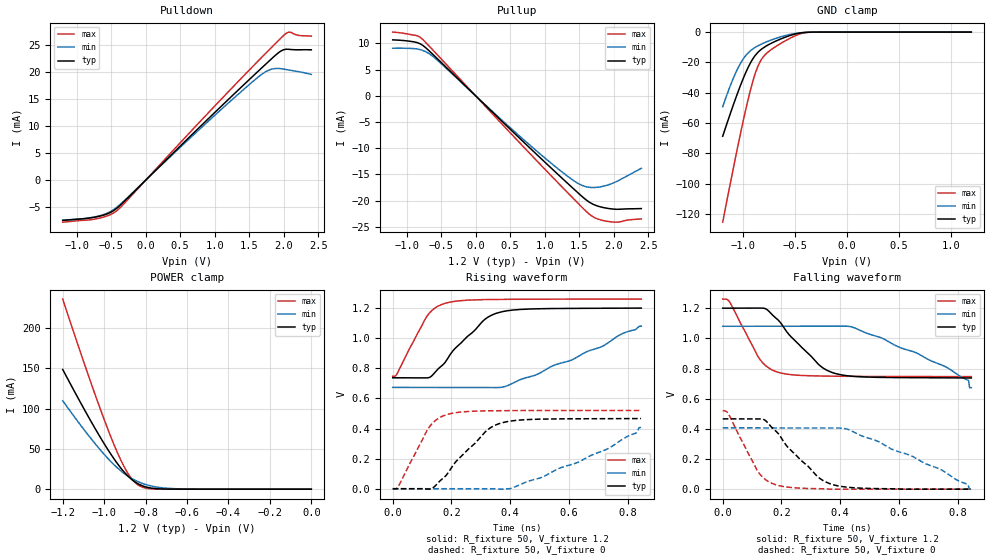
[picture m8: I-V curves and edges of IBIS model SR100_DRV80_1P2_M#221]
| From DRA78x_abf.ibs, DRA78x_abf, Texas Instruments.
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| Model based on original model for DDR_DIFFIOPB_V
|   Sub model SR100_DRV80_1P2
[model]   SR100_DRV80_1P2_M#221
|[Description]  [1.2V-I/O-X-X]
|   , ,
|[Input Load]
|[Output Drive]
|Voltage   1.2V
|Mode   I/O
Model_type   I/O
Polarity   Non-Inverting
Enable   Active-Low
Vinl =  0.47
Vinh =  0.73
Cref =  15.0000pF
Rref =  100.0000M
Vref =  0V
Vmeas =  0.6
C_comp   2p   2p   2p
[Model Spec]
Vinl   0.47   0.41   0.50
Vinh   0.73   0.67   0.76
[Receiver Thresholds]
Tslew_ac = 5n
Vth = 0.6
Vth_max = 0.63
Vth_min = 0.54
Vinh_ac = 0.22
Vinh_dc = 0.13
Vinl_ac = -0.22
Vinl_dc = -0.13
[Temperature Range]   25   125   -40
[Voltage Range]   1.2   1.08   1.26
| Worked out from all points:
|   slope of the pulldown table from 0 to 0.18 V, typ, clamps not added: 79.2 ohm
|   slope of the pullup table from 0 to 0.18 V, typ, clamps not added: 78.2 ohm
|   GND clamp passes 1 mA (typ) near -0.48 V on its own axis
|   POWER clamp passes 1 mA (typ) near -0.76 V on its own axis
|   rising waveform, R_fixture 50, V_fixture 1.2: 20-80 % time 130ps typ, 268ps min, 84.1ps max; typ from 0.737 V to 1.2 V
|   rising waveform, R_fixture 50, V_fixture 0: 20-80 % time 129ps typ, 266ps min, 84.2ps max; typ from 0 V to 0.466 V
|   falling waveform, R_fixture 50, V_fixture 1.2: 20-80 % time 130ps typ, 258ps min, 84.7ps max; typ from 1.2 V to 0.737 V
|   falling waveform, R_fixture 50, V_fixture 0: 20-80 % time 131ps typ, 262ps min, 83.9ps max; typ from 0.466 V to 0 V
[POWER_clamp]
-1.2V     148.6mA    109.7mA    235.9mA
-1.115V   108mA      79.97mA    170.5mA
-1.055V   80.16mA    59.93mA    125.3mA
-1.006V   59.04mA    45.03mA    90.73mA
-957.6mV  39.59mA    31.69mA    58.49mA
-921.2mV  26.75mA    23.11mA    36.96mA
-897mV    19.41mA    18.26mA    24.7mA
-860.6mV  10.74mA    12.35mA    10.83mA
-836.4mV  6.696mA    9.316mA    5.268mA
-787.9mV  2.052mA    4.939mA    818.3uA
-666.7mV  49.08uA    692.2uA    5.202uA
0V        48.89nA    205.6nA    269.9nA
[Pulldown]
-1.2V     -7.405mA   -7.369mA   -7.736mA
-690.9mV  -6.7mA     -6.627mA   -7.049mA
-509.1mV  -5.944mA   -5.774mA   -6.338mA
-400mV    -4.987mA   -4.803mA   -5.44mA
1.018V    12.71mA    12.18mA    13.93mA
1.527V    18.9mA     17.95mA    20.68mA
1.745V    21.5mA     20.08mA    23.52mA
1.855V    22.78mA    20.59mA    24.92mA
1.964V    23.89mA    20.6mA     26.3mA
2.073V    24.18mA    20.36mA    27.36mA
2.218V    24.09mA    20.04mA    26.74mA
2.4V      24.09mA    19.54mA    26.61mA
[Pullup]
-1.2V     10.67mA    9.076mA    12.16mA
-836.4mV  10.12mA    8.913mA    11.42mA
-763.6mV  9.612mA    8.654mA    10.74mA
-654.5mV  8.359mA    7.881mA    9.24mA
836.4mV   -10.59mA   -9.996mA   -11.72mA
1.273V    -15.99mA   -14.76mA   -17.69mA
1.527V    -19.06mA   -17.03mA   -21.1mA
1.6V      -19.87mA   -17.37mA   -22.05mA
1.709V    -20.76mA   -17.52mA   -23.17mA
1.855V    -21.36mA   -17.25mA   -23.85mA
2.036V    -21.67mA   -16.4mA    -24.14mA
2.4V      -21.54mA   -13.85mA   -23.51mA
[GND_clamp]
-1.2V     -68.74mA   -49.24mA   -125.5mA
-1.127V   -53.92mA   -35.5mA    -100.1mA
-1.055V   -39.92mA   -23.99mA   -75.5mA
-981.8mV  -27.37mA   -15.83mA   -52.4mA
-909.1mV  -17.63mA   -11.09mA   -32.41mA
-860.6mV  -13.38mA   -9.079mA   -22.59mA
-836.4mV  -11.86mA   -8.241mA   -19.18mA
-787.9mV  -9.515mA   -6.746mA   -14.76mA
-739.4mV  -7.652mA   -5.419mA   -11.95mA
-521.2mV  -1.657mA   -1.168mA   -3.09mA
-375.8mV  -108.2uA   -128.9uA   -198.1uA
1.2V      48.89nA    308.5nA    224.4nA
[Ramp]
dV/dt_f 0.27814318/0.12974707n 0.24489721/0.25925012n 0.30866525/84.85737p
dV/dt_r 0.28137411/0.12940691n 0.24550606/0.26785726n 0.31386717/84.489571p
R_load = 50
[Rising Waveform]
R_fixture = 50
V_fixture = 1.2
V_fixture_min = 1.08
V_fixture_max = 1.26
0s        737.2mV    673mV      747.1mV
14.4ps    737mV      672.9mV    762.3mV
118.2ps   736.5mV    672.9mV    1.15V
142.5ps   769.9mV    672.9mV    1.199V
175.6ps   832.6mV    673mV      1.23V
207.5ps   922.2mV    672.8mV    1.244V
308.2ps   1.116V     672.7mV    1.256V
367.6ps   1.174V     673.1mV    1.258V
607.4ps   1.198V     853.5mV    1.26V
846.3ps   1.2V       1.08V      1.26V
[Rising Waveform]
R_fixture = 50
V_fixture = 0
V_fixture_min = 0
V_fixture_max = 0
0s        0V         0V         0V
19.8ps    0V         0V         17.35mV
126ps     -2.385mV   0V         413.9mV
182.1ps   89.35mV    0V         491.5mV
311.6ps   371.2mV    0V         517.3mV
362.4ps   432.4mV    -2.208mV   518.5mV
399.1ps   449mV      0V         519mV
627.5ps   464.8mV    173mV      519.9mV
735.4ps   465.4mV    268.9mV    520mV
845.3ps   466.2mV    406.3mV    520mV
[Falling Waveform]
R_fixture = 50
V_fixture = 1.2
V_fixture_min = 1.08
V_fixture_max = 1.26
0s        1.2V       1.08V      1.26V
26ps      1.2V       1.08V      1.233V
131.1ps   1.201V     1.08V      848.9mV
187.5ps   1.124V     1.08V      775.4mV
325.9ps   827.8mV    1.08V      750.5mV
378.6ps   769.5mV    1.08V      748.9mV
441.7ps   748.4mV    1.074V     748mV
656.7ps   739.1mV    905.8mV    746.7mV
836.9ps   738.1mV    720.8mV    746.4mV
846.3ps   737.2mV    673mV      746.4mV
[Falling Waveform]
R_fixture = 50
V_fixture = 0
V_fixture_min = 0
V_fixture_max = 0
0s        466.2mV    406.3mV    519.6mV
19.9ps    466.3mV    406.4mV    498.9mV
120.7ps   466.3mV    406.4mV    114.7mV
143.6ps   457.7mV    406.4mV    66.76mV
175.5ps   394mV      406.4mV    32.33mV
321.6ps   85.87mV    406.4mV    2.92mV
375.5ps   29.52mV    406.5mV    0V
427.4ps   12.26mV    395.7mV    0V
641.6ps   0V         221.7mV    0V
845.3ps   0V         0V         0V
